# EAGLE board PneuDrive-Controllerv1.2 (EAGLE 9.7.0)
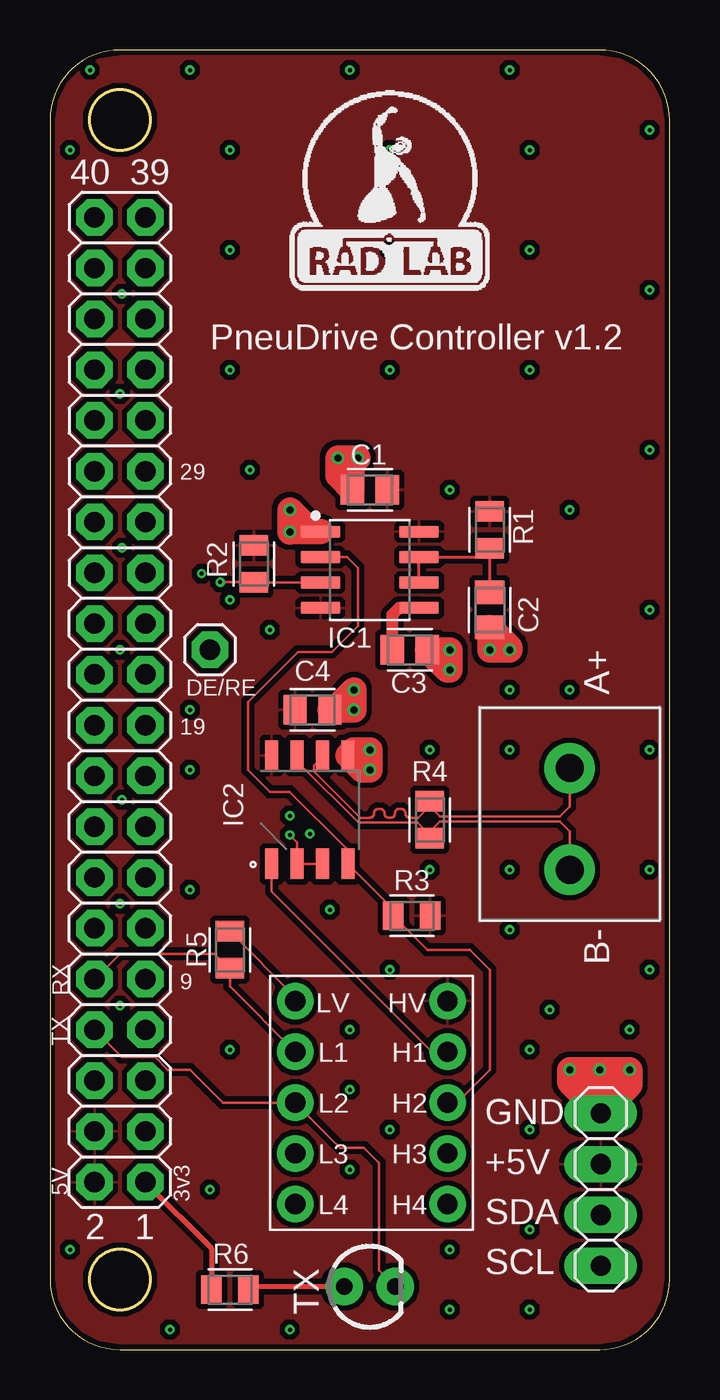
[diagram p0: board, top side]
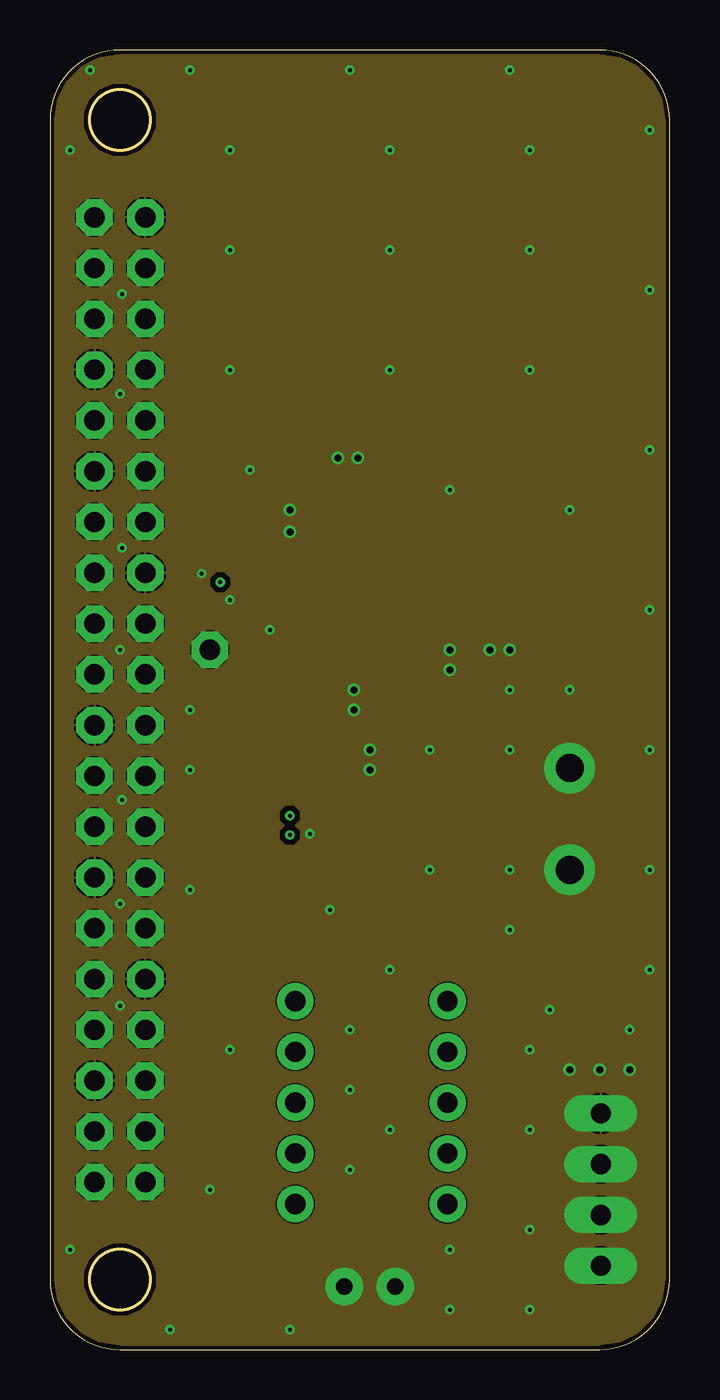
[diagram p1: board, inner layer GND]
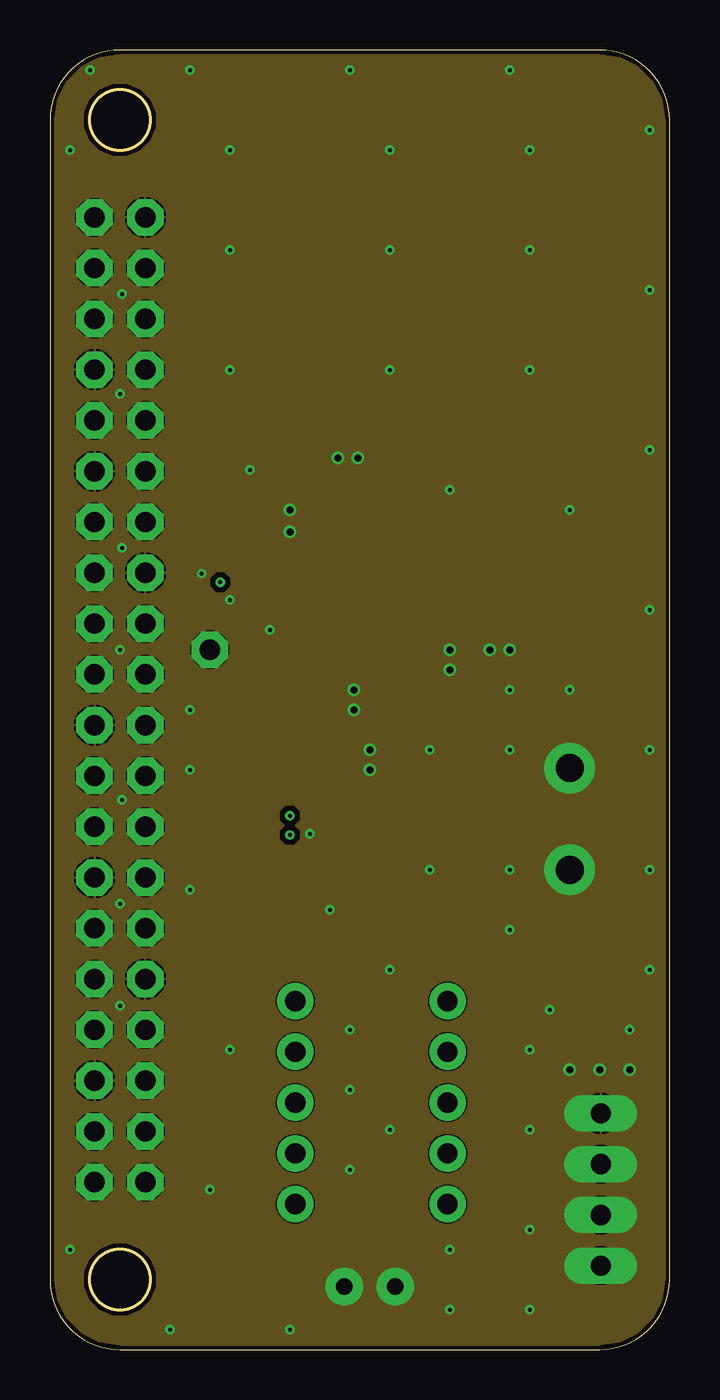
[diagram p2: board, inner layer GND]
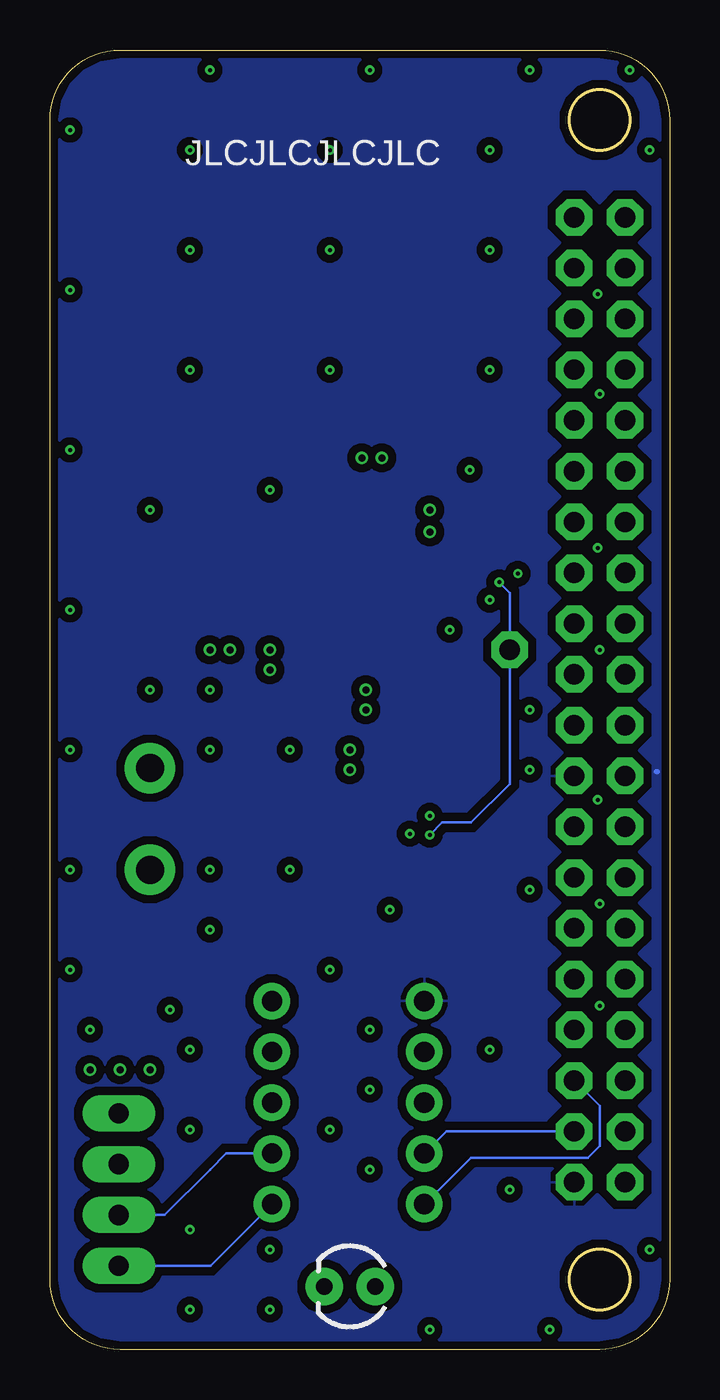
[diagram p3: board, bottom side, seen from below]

Size 31 x 65 mm. Coordinates in mm from the lower left corner, seen from the top.
Outline: 31,3.5 31,61.5 arc90 27.5,65 3.5,65 arc90 0,61.5 0,3.5 arc90 3.5,0 27.5,0 arc90 31,3.5
Outline: circle at 3.5,3.5 radius 1.5
Outline: circle at 3.5,61.5 radius 1.5
Copper layers (1+2*15+16): Top / GND / GND / Bottom
Stack-up Default Layer Stack: Top User Defined 0.035mm / Dielectric-2 User Defined 0.2mm / GND User Defined 0.0175mm / Dielectric-1 User Defined 1.065mm / GND User Defined 0.0175mm / Dielectric-3 User Defined 0.2mm / Bottom User Defined 0.035mm
Design rules: minimum copper width class=2 0.116840625mm, minimum copper width 3.5mil, minimum drill size 0.2mm, copper clearance via to via 0.5mm, copper clearance wire_polygon to via 10mil, copper clearance class=2 to class=1 8mil, copper clearance class=2 to class=0 8mil, copper clearance wire_polygon to pad_smd 0.2mm, copper clearance wire_polygon to wire_polygon 5mil, copper clearance pad_smd to pad_smd 5mil, copper clearance pad_smd to via 5mil, copper clearance smd to pad (same net) 5mil, copper clearance smd to via (same net) 5mil, copper clearance smd to smd (same net) 5mil, dimension clearance 0.2mm, restrict clearance 0mil, drill distance 6mil, keepout clearance 0mil
Net classes: 2 impedance_120: width 0.117 mm, clearance 0.203 mm to class 0, clearance 0.203 mm to class 1

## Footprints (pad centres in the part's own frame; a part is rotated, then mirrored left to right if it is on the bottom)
CAPC2012X110 = smd 1.165 x 1.465: 1 -0.875,0; 2 0.875,0
SOIC127P599X175-8N = smd 1.965 x 0.602: 1 -2.47,1.905; 2 -2.47,0.635; 3 -2.47,-0.635; 4 -2.47,-1.905; 5 2.47,-1.905; 6 2.47,-0.635; 7 2.47,0.635; 8 2.47,1.905
SOIC127P600X175-8N = smd 1.525 x 0.65: 1 -2.712,1.905; 2 -2.712,0.635; 3 -2.712,-0.635; 4 -2.712,-1.905; 5 2.712,-1.905; 6 2.712,-0.635; 7 2.712,0.635; 8 2.712,1.905
2828412 = drill 1.4 pad 2.1: 1 0,0; 2 5.08,0
2X20 = drill 1.016 octagon: 1 -24.13,-1.27; 2 -24.13,1.27; 3 -21.59,-1.27; 4 -21.59,1.27; 5 -19.05,-1.27; 6 -19.05,1.27; 7 -16.51,-1.27; 8 -16.51,1.27; 9 -13.97,-1.27; 10 -13.97,1.27; 11 -11.43,-1.27; 12 -11.43,1.27; 13 -8.89,-1.27; 14 -8.89,1.27; 15 -6.35,-1.27; 16 -6.35,1.27; 17 -3.81,-1.27; 18 -3.81,1.27; 19 -1.27,-1.27; 20 -1.27,1.27; 21 1.27,-1.27; 22 1.27,1.27; 23 3.81,-1.27; 24 3.81,1.27; 25 6.35,-1.27; 26 6.35,1.27; 27 8.89,-1.27; 28 8.89,1.27; 29 11.43,-1.27; 30 11.43,1.27; 31 13.97,-1.27; 32 13.97,1.27; 33 16.51,-1.27; 34 16.51,1.27; 35 19.05,-1.27; 36 19.05,1.27; 37 21.59,-1.27; 38 21.59,1.27; 39 24.13,-1.27; 40 24.13,1.27
1X04 = drill 1.016 long: 1 -3.81,0; 2 -1.27,0; 3 1.27,0; 4 3.81,0
1X01 = drill 1.016 octagon: 1 0,0
RESC2012X65 = smd 1.031 x 1.42: 1 -0.919,0; 2 0.919,0
POLOLU_LOGIC_SHIFTER = drill 1.016: 1 1.27,11.43; 2 1.27,8.89; 3 1.27,6.35; 4 1.27,3.81; 5 1.27,1.27; 6 8.89,1.27; 7 8.89,3.81; 8 8.89,6.35; 9 8.89,8.89; 10 8.89,11.43
LED_3MM = drill 0.813 pad 1.88: A -1.27,0; K 1.27,0

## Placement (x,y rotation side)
C1  .1uF  [CAPC2012X110]  16,43 180 top
C2  .1u  [CAPC2012X110]  22,37 270 top
C3  10n  [CAPC2012X110]  18,35 0 top
C4  .1uF  [CAPC2012X110]  13.14,32 0 top
IC1  LM555_SOIC  [SOIC127P599X175-8N]  16,39 0 top
IC2  THVD1428  [SOIC127P600X175-8N]  13,27 90 top
J1  282841-2  [2828412]  26,24 90 top
JP1  [2X20]  3.5,32.5 90 top
JP2  [1X04]  27.56,8 270 top
JP4  [1X01]  8,35 0 top
R1  1k  [RESC2012X65]  22,41 90 top
R2  10k  [RESC2012X65]  10.2,39.3 270 top
R3  4.3k  [RESC2012X65]  18.1,21.7 0 top
R4  120  [RESC2012X65]  19,26.5 270 top
R5  4.3k  [RESC2012X65]  9,20 90 top
R6  732  [RESC2012X65]  9,3 180 top
SHIFTER1  POLOLU_LOGIC_SHIFTERPOLOLU  [POLOLU_LOGIC_SHIFTER]  11,6 0 top
TX  Green  [LED_3MM]  16,3.15 0 top

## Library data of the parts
C1-C4 = Capacitor; CATEGORY: Capacitor
IC1 = IC_Clock-Timing; CATEGORY: IC_Clock-Timing; CURRENT-SUPPLY: 10mA; DESCRIPTION: IC OSC SGL TIMER 100KHZ 8-SOIC; FREQUENCY: 100kHz; MANUFACTURER: Texas Instruments; MPN: LM555CM/NOPB; OPERATING_TEMP: 0°C to 70°C; PART_STATUS: Active; ROHS_COMPLIANT: ROHS3 Compliant; SUB-CATEGORY: Timer
IC2 = Library; DESCRIPTION: RS-485 Interface IC; HEIGHT: 1.75mm; MANUFACTURER_NAME: Texas Instruments; MANUFACTURER_PART_NUMBER: SN65HVD08DR; MOUSER_PART_NUMBER: 595-SN65HVD08DR; MOUSER_PRICE-STOCK: https://www.mouser.com/ProductDetail/Texas-Instruments/SN65HVD08DR?qs=QViXGNcIEAtwhwZ8YvgaIA%3D%3D
J1 = Library; DESCRIPTION: TERMI-BLOK PCB MOUNT 2P. 5; HEIGHT: 15.45mm; MANUFACTURER_NAME: TE Connectivity; MANUFACTURER_PART_NUMBER: 282841-2; MOUSER_PART_NUMBER: 571-2828412; MOUSER_PRICE-STOCK: https://www.mouser.co.uk/ProductDetail/TE-Connectivity/282841-2?qs=gdajpSf3VLd4K34xU%252BwLgw%3D%3D
JP1 JP2 JP4 = pinhead
R1-R6 = Resistor; CATEGORY: Resistor; SUB-CATEGORY: Fixed
SHIFTER1 = Library
TX = SparkFun-LED; PROD_ID: DIO-08794

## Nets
3V3: JP1.1 JP1.17 R5.2 R6.2 SHIFTER1.1
+5V: C1.1 C4.1 IC1.4 IC1.8 IC2.8 JP1.2 JP1.4 JP2.2 R1.2 R2.1 R3.2 SHIFTER1.10
CV: C3.1 IC1.5
DE/RE: IC1.3 IC2.2 IC2.3 JP4.1 R2.2
GND: C1.2 C2.2 C3.2 C4.2 IC1.1 IC2.5 JP1.6 JP1.9 JP1.14 JP1.20 JP1.25 JP1.30 JP1.34 JP1.39 JP2.1
I2C_SCL_3V3: JP1.5 SHIFTER1.5
I2C_SCL_5V: JP2.4 SHIFTER1.6
I2C_SDA_3V3: JP1.3 SHIFTER1.4
I2C_SDA_5V: JP2.3 SHIFTER1.7
N$1: R6.1 TX.A
RX_3V3: JP1.10 R5.1 SHIFTER1.2
RX_5V: IC2.1 SHIFTER1.9
SER_N [impedance_120]: IC2.7 J1.1 R4.2
SER_P [impedance_120]: IC2.6 J1.2 R4.1
THRESH: C2.1 IC1.6 IC1.7 R1.1
TX_3V3: JP1.8 SHIFTER1.3 TX.K
TX_5V: IC1.2 IC2.4 R3.1 SHIFTER1.8

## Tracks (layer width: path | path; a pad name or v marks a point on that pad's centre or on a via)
3V3
  Top 0.127: R5.2 12.27,17.65 SHIFTER1.1
  Top 0.254: JP1.1 8.08,5.06 R6.2
  Bottom 0.254: 0.6,28.9 0.68,28.9
  pour Bottom (isolate 0.406): 0,0 0,65 31,65 31,0
+5V
  pour Top (isolate 0.254): 0,0 31,0 31,65 0,65
CV
  Top 0.61: IC1.5 17.47,37.09 17.12,36.75 C3.1
DE/RE  (via drill 0.2)
  Top 0.127: IC2.3 IC2.2 12.37,25.38 v12,25.74 | IC1.3 10.22,38.37 R2.2 8.54,38.38 v8.52,38.38
  Bottom 0.127: v8.52,38.38 8.52,38.36 8,37.84 JP4.1 8,28.3 9.94,26.36 11.38,26.36 v12,25.74
GND  (via drill 0.2, 0.35)
  Top 1.27: v26,14 27.56,12.44 JP2.1 | JP2.1 27.56,13.94 v27.5,14 | JP2.1 27.56,12.56 v29,14 | v29,14 v26,14 | JP2.1 26,13.37 v26,14 | JP2.1 29,13.25 v29,14 | C1.2 15.12,44.33 v15.4,44.6 v14.4,44.6 | C1.2 15.12,43.88 v14.4,44.6 | v14.4,44.6 14.4,43.73 C1.2 | v12,42 13.1,40.91 IC1.1 v12.01,40.91 v12,40.9 v12,42 | C2.2 v22,35 v23,35 23,35.12 C2.2 | C3.2 v20,35 v20,34 19.88,34 C3.2 | C4.2 v15.2,32 v15.2,33 14.2,32 C4.2 | IC2.5 15.19,30 v16,30 v16,29 15.62,29 IC2.5
  other vias: 9,37.5 7.59,38.81 8,8 15,16 15,13 15,9 17,11 20,2 20,5 24,2 24,6 24,11 24,15 25,17 30,19 29,16 19,24 23,24 23,21 23,30 19,30 23,33 26,33 30,30 30,24 7,29 7,32 11,36 30,37 30,45 30,53 30,61 23,64 15,64 7,64 2,64 1,60 9,60 9,55 9,49 17,49 17,60 24,49 24,60 24,55 17,55 10,44 20,43 26,42 1,5 3.5,22.3 3.6,27.5 3.5,17.2 6,1 12,1 14,22 17,19 3.6,52.8 3.5,47.8 3.6,40.1 3.5,35 9,15 7,23 13,25.8
  pour GND: 0,0 31,0 31,65 0,65
  pour GND: 0,0 31,0 31,65 0,65
GND1  (via drill 0.2)
  other vias: 12,26.7
I2C_SCL_3V3
  Bottom 0.127: JP1.5 3.5,12.18 3.5,10.2 4.1,9.6 6.9,9.6 9.94,9.6 SHIFTER1.5
I2C_SCL_5V
  Bottom 0.127: SHIFTER1.6 22.97,4.19 JP2.4
I2C_SDA_3V3
  Bottom 0.127: JP1.3 11.17,10.91 SHIFTER1.4
I2C_SDA_5V
  Bottom 0.127: SHIFTER1.7 22.19,9.81 23,9 25.27,6.73 JP2.3
N$1
  Top 0.254: R6.1 10.07,3.15 TX.A
RX_3V3
  Top 0.127: JP1.10 3.5,19.8 5.8,19.8 8.2,19.8 8.92,19.08 | SHIFTER1.2 9,18.16 R5.1
  Top 0.152: 8.92,19.08 R5.1
RX_5V
  Top 0.127: IC2.1 11.1,22.91 19.11,14.89 SHIFTER1.9
SER_N
  Top 0.117: J1.1 26,25.92 25.5,26.42 19.5,26.42 19,25.92 R4.2 18.88,25.46 19,25.33 19,25.73 18.38,26.36 18,26.36 16,26.36 15.43,26.36 12.56,29.22 12.56,29.51 IC2.7
SER_P
  Top 0.117: J1.2 26,27.16 25.5,26.66 19.5,26.66 19,27.16 R4.1 19,27.2 18.4,26.6 18,26.6 arc-90 17.78,26.82 17.78,26.83 arc90 17.57,27.04 17.48,27.04 arc90 17.26,26.83 17.26,26.82 arc-90 17.04,26.6 16.96,26.6 arc-90 16.74,26.82 16.74,26.83 arc90 16.52,27.04 16.43,27.04 arc90 16.22,26.83 16.22,26.82 arc-90 16,26.6 15.53,26.6 13.22,28.91 13.22,29.2 13.63,29.62 IC2.6
THRESH
  Top 0.152: C2.1 R1.1 21.55,39.63 IC1.7 IC1.6
TX_3V3
  Top 0.127: JP1.8 3.59,14.63 5.26,14.63 5.89,14 7,14 8.65,12.35 SHIFTER1.3 14.52,10.1 15.7,10.1 16.47,9.33 16.47,3.95 TX.K
TX_5V
  Top 0.127: IC1.2 14.87,39.63 15.4,39.1 15.4,36.2 14.1,34.9 12.4,34.9 9.9,32.4 9.9,29 11,27.9 11.98,27.9 14.8,25.08 14.8,24.39 IC2.4 17.18,22.01 R3.1 18.88,20 21,20 22,19 22,14 20.35,12.35 SHIFTER1.8

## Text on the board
tPlace: 40 | 39 | PneuDrive Controller v1.2 | 29 | DE/RE | A+ | 19 | B- | RX | 9 | TX | GND | +5V | 5V | 3v3 | 2 | 1 | SDA | SCL
bPlace: JLCJLCJLCJLC

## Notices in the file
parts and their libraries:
SparkFun-LED: Licensing: Creative Commons ShareAlike 4.0 International - https://creativecommons.org/licenses/by-sa/4.0
